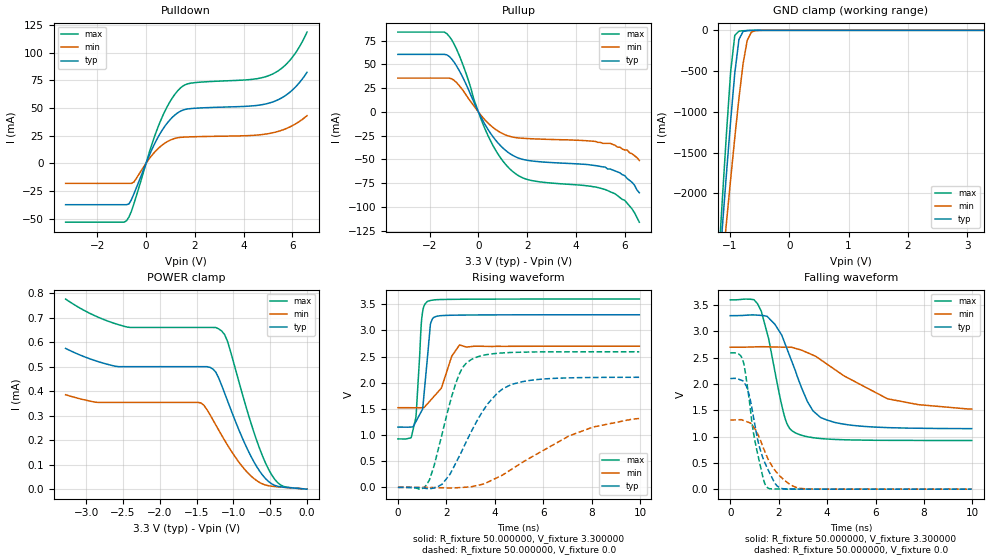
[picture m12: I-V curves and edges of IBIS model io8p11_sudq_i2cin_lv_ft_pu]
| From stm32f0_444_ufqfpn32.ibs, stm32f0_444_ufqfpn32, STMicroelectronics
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|   Model io8p11_sudq_i2cin_lv_ft_pu
[Model]  io8p11_sudq_i2cin_lv_ft_pu
Model_type I/O
Polarity   Non-Inverting
Enable   Active-Low
Vinl =   0.990000V
Vinh =   2.310000V
Vmeas =  1.650000V
Cref =   30.000000pF
Rref =   100.000000M
Vref =   0.0V
C_comp   2.070000pF   1.996000pF   2.160200pF
[Temperature Range]   25.000000   0.125000k   -40.000000
[Pullup Reference]   3.300000V   2.700000V   3.600000V
[Pulldown Reference]   0.0V   0.0V   0.0V
[POWER Clamp Reference]   3.300000V   2.700000V   3.600000V
[GND Clamp Reference]   0.0V   0.0V   0.0V
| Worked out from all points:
|   slope of the pulldown table from 0 to 0.495 V, typ, clamps not added: 20.9 ohm
|   slope of the pullup table from 0 to 0.495 V, typ, clamps not added: 22.2 ohm
|   GND clamp passes 1 mA (typ) near -0.64 V on its own axis
|   rising waveform, R_fixture 50.000000, V_fixture 3.300000: 20-80 % time 255ps typ, 664ps min, 194ps max; typ from 1.15 V to 3.3 V
|   rising waveform, R_fixture 50.000000, V_fixture 0.0: 20-80 % time 1.54ns typ, 3.06ns min, 906ps max; typ from 0.001 V to 2.1 V
|   falling waveform, R_fixture 50.000000, V_fixture 3.300000: 20-80 % time 1.12ns typ, 2.6ns min, 729ps max; typ from 3.3 V to 1.15 V
|   falling waveform, R_fixture 50.000000, V_fixture 0.0: 20-80 % time 673ps typ, 889ps min, 535ps max; typ from 2.1 V to 0.001 V
[Pulldown]
|Voltage   I(typ)   I(min)   I(max)
-3.3V     -37.45mA   -18.2mA    -53.24mA
-800mV    -37.45mA   -18.2mA    -51.9mA
-700mV    -36.7mA    -18.2mA    -48.48mA
-500mV    -27.71mA   -17.01mA   -36.66mA
500mV     23.91mA    13.38mA    33.24mA
900mV     37.17mA    19.88mA    52.48mA
1.3V      45.55mA    23.01mA    65.5mA
1.8V      49.29mA    23.83mA    72.18mA
4.4V      51.88mA    25.21mA    75.91mA
5.2V      55.41mA    27.53mA    80.72mA
5.9V      64.2mA     32.82mA    93.01mA
6.6V      82.13mA    42.97mA    118.5mA
[Pullup]
|Voltage   I(typ)   I(min)   I(max)
-3.3V     60.63mA    35.66mA    84.09mA
-1.4V     60.63mA    35.66mA    84.09mA
-1.2V     58.55mA    35.66mA    79.71mA
-700mV    39.46mA    25.05mA    54.09mA
-100mV    5.36mA     3.465mA    7.201mA
400mV     -18.61mA   -11.78mA   -25.23mA
900mV     -35.28mA   -21.54mA   -48mA
1.5V      -46.91mA   -26.86mA   -64.57mA
2.2V      -51.57mA   -28.22mA   -72.25mA
5.3V      -60mA      -33mA      -82.7mA
6V        -67mA      -40mA      -93mA
6.6V      -85mA      -51mA      -116mA
[GND_clamp]
|Voltage   I(typ)   I(min)   I(max)
-3.3V     -9.366A    -9.678A    -9.859A
-1.2V     -3.091A    -3.431A    -2.911A
-1.13V    -2.415A    -2.888A    -2.072A
-1.06V    -1.751A    -2.352A    -1.259A
-990mV    -1.112A    -1.826A    -509.3mA
-920mV    -522.9mA   -1.315A    -61.61mA
-850mV    -112.5mA   -833.8mA   -10.22mA
-780mV    -13.59mA   -408.1mA   -5.256mA
-710mV    -3.081mA   -122.1mA   -2.635mA
-640mV    -945.2uA   -21.36mA   -905.7uA
-570mV    -199.6uA   -4.142mA   -156.8uA
3.28V     0A         0A         0A
[POWER_clamp]
|Voltage   I(typ)   I(min)   I(max)
-3.28V    574uA      385.1uA    775.2uA
-2.88V    524.3uA    354.9uA    706.9uA
-2.44V    499.5uA    353.8uA    660.7uA
-1.44V    499.5uA    351.5uA    659.5uA
-1.28V    490.2uA    283.5uA    659.5uA
-1.16V    423.6uA    220uA      645uA
-1.08V    360.3uA    179.6uA    602.6uA
-800mV    157uA      65.19uA    307.1uA
-640mV    71.83uA    26.55uA    162.4uA
-520mV    30.52uA    13.8uA     79.51uA
-360mV    9.625uA    8.656uA    17.31uA
0V        0A         0A         0A
[Ramp]
| variable   typ   min   max
dV/dt_r  1.26168/1.53431n   0.74146/3.04310n   1.55427/0.90477n
dV/dt_f  1.28748/1.11982n   0.68808/2.60012n   1.60394/0.72751n
R_load = 50.000000
[Rising Waveform]
R_fixture= 50.000000
V_fixture= 3.300000
V_fixture_min= 2.700000
V_fixture_max= 3.600000
|time   V(typ)   V(min)   V(max)
0s        1.152V     1.524V     926.8mV
540.5ps   1.154V     1.523V     947.3mV
740.7ps   1.257V     1.522V     1.337V
981ps     1.464V     1.523V     3.221V
1.221ns   2.497V     1.6V       3.555V
1.341ns   3.117V     1.662V     3.572V
1.441ns   3.234V     1.714V     3.581V
1.802ns   3.284V     1.905V     3.591V
2.543ns   3.293V     2.722V     3.596V
9.97ns    3.3V       2.7V       3.6V
[Rising Waveform]
R_fixture= 50.000000
V_fixture= 0.0
V_fixture_min= 0.0
V_fixture_max= 0.0
|time   V(typ)   V(min)   V(max)
0s        1.088mV    1.198mV    1.045mV
1.181ns   -22mV      212uV      46.59mV
1.481ns   -10.79mV   -2.923mV   396.1mV
1.822ns   59.65mV    -7.882mV   1.019V
2.382ns   459.6mV    -7.896mV   1.977V
3.003ns   1.042V     12.21mV    2.437V
3.724ns   1.605V     103.9mV    2.542V
4.765ns   1.977V     367.9mV    2.58V
7.067ns   2.093V     984.3mV    2.591V
9.97ns    2.105V     1.317V     2.592V
[Falling Waveform]
R_fixture= 50.000000
V_fixture= 3.300000
V_fixture_min= 2.700000
V_fixture_max= 3.600000
|time   V(typ)   V(min)   V(max)
0s        3.3V       2.7V       3.6V
981ps     3.314V     2.706V     3.602V
1.281ns   3.304V     2.71V      3.382V
1.842ns   3.137V     2.703V     2.243V
2.202ns   2.838V     2.701V     1.449V
2.663ns   2.285V     2.682V     1.079V
3.403ns   1.499V     2.552V     980.9mV
3.984ns   1.318V     2.383V     955.1mV
6.486ns   1.172V     1.721V     929.6mV
9.97ns    1.152V     1.524V     926.8mV
[Falling Waveform]
R_fixture= 50.000000
V_fixture= 0.0
V_fixture_min= 0.0
V_fixture_max= 0.0
|time   V(typ)   V(min)   V(max)
0s        2.105V     1.317V     2.592V
340.3ps   2.093V     1.321V     2.573V
560.6ps   2.035V     1.305V     2.386V
760.8ps   1.825V     1.271V     1.776V
1.021ns   1.214V     1.145V     914.6mV
1.381ns   558mV      767.8mV    171.3mV
1.562ns   369.9mV    572.1mV    22.41mV
2.042ns   26.26mV    253.8mV    3.402mV
2.903ns   3.01mV     15.94mV    2.004mV
9.97ns    1.088mV    1.198mV    1.045mV
